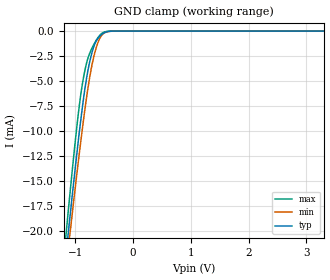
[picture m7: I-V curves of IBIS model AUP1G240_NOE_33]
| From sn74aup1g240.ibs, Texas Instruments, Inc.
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[Model]   AUP1G240_NOE_33
Model_type  Input
Vinl=0.9
Vinh=2
| variable   typ   min   max
C_comp   1.60pF   1.32pF   1.97pF
[Temperature Range]   40   100   -40
| Ambient temperature   25   85   -40
[Voltage range]   3.3   3   3.6
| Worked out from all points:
|   GND clamp passes 1 mA (typ) near -0.64 V on its own axis
[GND Clamp]
| AUP1G240_NOE_33
|   Voltage   I(typ)   I(min)   I(max)
-3.6V     -171.6mA   -163.5mA   -181.1mA
-1.16V    -22.22mA   -23.69mA   -20.18mA
-1.11V    -19.45mA   -21.09mA   -17.19mA
-1.085V   -18.08mA   -19.81mA   -15.71mA
-940mV    -10.5mA    -12.6mA    -7.822mA
-890mV    -8.117mA   -10.26mA   -5.698mA
-835mV    -5.768mA   -7.825mA   -3.925mA
-755mV    -3.153mA   -4.717mA   -2.255mA
-675mV    -1.463mA   -2.419mA   -1.277mA
-595mV    -617.7uA   -945.8uA   -546.7uA
-515mV    -215.4uA   -248.8uA   -134.4uA
3.3V      132.2pA    540.4pA    36.28pA
